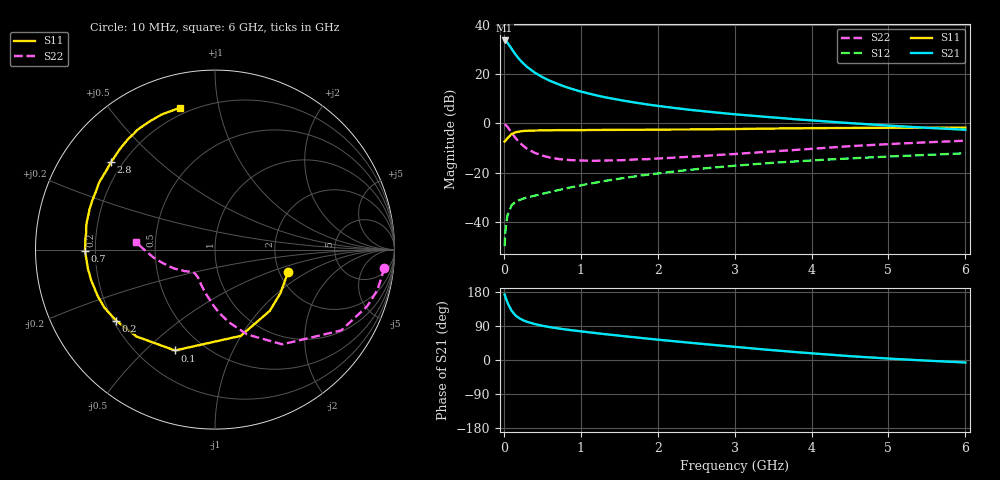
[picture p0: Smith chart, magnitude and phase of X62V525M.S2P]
! SIEMENS Small Signal Semiconductors
! BFP193W
! Si NPN RF Bipolar Junction Transistor in SOT343
! VCE = 2.5 V  IC = 25 mA
! Common Emitter S-Parameters:  April 1994
# GHz  S  MA  R  50
!  f  S11  S21  S12  S22
! GHz  MAG  ANG  MAG  ANG  MAG  ANG  MAG  ANG
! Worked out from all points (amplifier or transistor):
!   40 points, 10 MHz to 6 GHz, reference 50 ohm
!   highest |S21| = 33.6 dB at 10 MHz (marker M1)
!   |S21| within 3 dB of that: start of sweep to 92.7 MHz
!   unconditionally stable (mu >= 1): 840.3 MHz to 3.973 GHz
!   at 200 MHz: K = 0.41, MSG = 28.6 dB, |S12| = -31.2 dB
!   at 1.5 GHz: K = 1.12, MAG = 13.9 dB, |S12| = -22.5 dB
!   at 6 GHz: K = 0.95, MSG = 4.8 dB, |S12| = -12.2 dB
!   S11 on the Smith chart (normalised r, x): 10 MHz: 2.24, -0.67; 100 MHz: 0.35, -0.62; 200 MHz: 0.21, -0.31; 700 MHz: 0.16, -0.00; 2.8 GHz: 0.16, +0.36; 6 GHz: 0.16, +0.77
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0.01  0.4262 -16.8  47.85 172.7  0.0032 85.2  0.9494 -6.1
0.02  0.4375 -33.4  47.27 167.1  0.0063 78.1  0.9331 -13.9
0.03  0.4579 -48.1  46.08 161.2  0.0092 74.0  0.9048 -20.4
0.05  0.5017 -73.4  42.41 150.0  0.014 65.1  0.8352 -32.6
0.1  0.6045 -111.6  32.6 130.3  0.0215 50.3  0.6475 -54.6
0.15  0.6528 -132.2  25.11 117.9  0.0255 43.2  0.5055 -69.3
0.2  0.678 -144.3  19.96 110.3  0.0276 41.0  0.4116 -79.2
0.25  0.6958 -152.2  16.55 104.9  0.0294 39.7  0.3507 -86.6
0.3  0.7025 -158.0  13.98 100.9  0.0311 40.2  0.3041 -92.6
0.4  0.7106 -165.9  10.7 94.9  0.0338 42.0  0.2509 -101.7
0.5  0.7159 -171.6  8.658 90.3  0.037 44.7  0.2205 -108.7
0.6  0.7184 -175.8  7.248 86.7  0.0401 46.9  0.201 -114.2
0.7  0.7246 -179.5  6.273 83.6  0.0436 49.1  0.1887 -118.5
0.9  0.725 175.1  4.885 78.1  0.0511 51.9  0.1776 -124.8
1.1  0.7284 170.4  4.026 73.2  0.0589 54.2  0.1734 -129.3
1.6  0.7347 160.3  2.798 62.0  0.0791 56.2  0.1794 -135.9
2.2  0.7462 149.9  2.057 49.8  0.1042 55.3  0.1994 -143.0
2.8  0.7575 140.0  1.628 38.4  0.1292 52.6  0.228 -149.6
3.2  0.7697 134.0  1.433 31.2  0.1451 50.1  0.2498 -154.9
4.5  0.8021 116.7  1.006 10.1  0.1934 41.4  0.3422 -172.1
5.5  0.8097 108.0  0.808 -1.7  0.2277 35.1  0.4104 178.1
6  0.8143 103.7  0.738 -6.6  0.2459 32.2  0.4422 174.3
